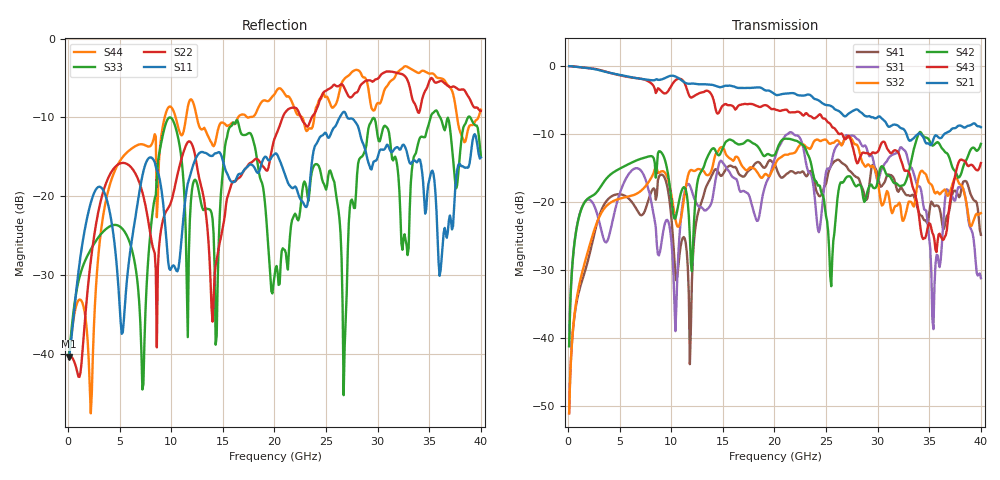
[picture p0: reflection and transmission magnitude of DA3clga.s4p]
! ADC12DJ3200QML-SP
! 196-pin ZMX package
! CLGA Ceramic Package without columns (ceramic land grid array)
! Texas Instruments 4/21/2021
! Single-ended  S-parameters
! PORT#  PORT_NAME  NET_NAME
! PORT1:  DAxN.DIEBUMP DAxN
! PORT2:  DAxN.BGA  DAxN
! PORT3:  DAxP.DIEBUMP DAxP
! PORT4:  DAxP.BGA  DAxP
! Touchstone Ver. 1.0
! Number of ports is 4
# Hz	S	MA	R	50.000000
! SCATTERING PARAMETERS  :
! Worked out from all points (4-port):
!   400 points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, 100 MHz to 40 GHz, reference 50 ohm
!   strongest paths, dB at 100 MHz, 10.1 GHz, 20.1 GHz, 30.1 GHz, 40 GHz:
!     S21: -0.1, -1.5, -4.3, -7.5, -9.1
!     S43: -0.1, -2.7, -6.5, -12.4, -14.3
!     S42: -41.3, -20.9, -12.9, -16.2, -11.5
!     S32: -51.1, -19.8, -14.4, -17.9, -21.7
!     S31: -41.3, -27.6, -13.3, -16.8, -31.3
!     S41: -51.1, -24.0, -14.7, -16.8, -24.9
!   lowest |S11| = -40.4 dB at 100 MHz (marker M1), VSWR 1.02, Z = 51 + j0.01 ohm
!   |S11| at or under -10 dB: start of sweep to 26.32 GHz; 27.05 GHz to end of sweep
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1e8  0.009563 0.6  0.9904 -3.8  0.008653 77.6  0.002781 -118.1
     0.9904 -3.8  0.009277 0.1  0.002777 -117.7  0.008642 79.7
     0.008653 77.6  0.002777 -117.7  0.009882 14.5  0.9905 -3.9
     0.002781 -118.1  0.008642 79.7  0.9905 -3.9  0.00978 13.9
4.8e9  0.03098 149.2  0.8607 -174.3  0.1022 91.5  0.1133 40.4
       0.8607 -174.3  0.1579 1.4  0.104 40.8  0.1714 27.2
       0.1022 91.5  0.104 40.8  0.06516 85.4  0.8561 -176.6
       0.1133 40.4  0.1714 27.2  0.8561 -176.6  0.1576 12.7
7.2e9  0.1346 -132.4  0.7967 103.8  0.1636 -34.4  0.08004 -55.1
       0.7967 103.8  0.1057 -81.4  0.1226 -51.9  0.2081 8.5
       0.1636 -34.4  0.1226 -51.9  0.00592 -74.8  0.7963 97.9
       0.08004 -55.1  0.2081 8.5  0.7963 97.9  0.213 -62.0
1.01e10  0.03593 -89.7  0.8429 3.4  0.04182 -25.3  0.06282 128.8
         0.8429 3.4  0.09757 -28.6  0.1023 161.4  0.09054 -35.7
         0.04182 -25.3  0.1023 161.4  0.3073 -10.7  0.7301 8.4
         0.06282 128.8  0.09054 -35.7  0.7301 8.4  0.3591 -124.0
2.67e10  0.3425 155.4  0.4284 134.7  0.2758 74.5  0.1892 -36.7
         0.4284 134.7  0.4966 -105.5  0.2795 -32.7  0.14 -4.0
         0.2758 74.5  0.2795 -32.7  0.005451 -49.0  0.2967 129.2
         0.1892 -36.7  0.14 -4.0  0.2967 129.2  0.5468 -81.1
2.95e10  0.1565 -1.1  0.4171 37.7  0.212 11.3  0.1861 -124.5
         0.4171 37.7  0.5314 -114.1  0.183 -157.0  0.1286 -7.8
         0.212 11.3  0.183 -157.0  0.3103 -30.9  0.23 50.8
         0.1861 -124.5  0.1286 -7.8  0.23 50.8  0.3532 -123.0
4e10  0.1757 105.3  0.3526 35.9  0.02736 112.4  0.05706 -139.0
      0.3526 35.9  0.3471 -166.1  0.08236 157.3  0.2658 -11.3
      0.02736 112.4  0.08236 157.3  0.1791 -154.1  0.1921 106.8
      0.05706 -139.0  0.2658 -11.3  0.1921 106.8  0.3536 -148.4
